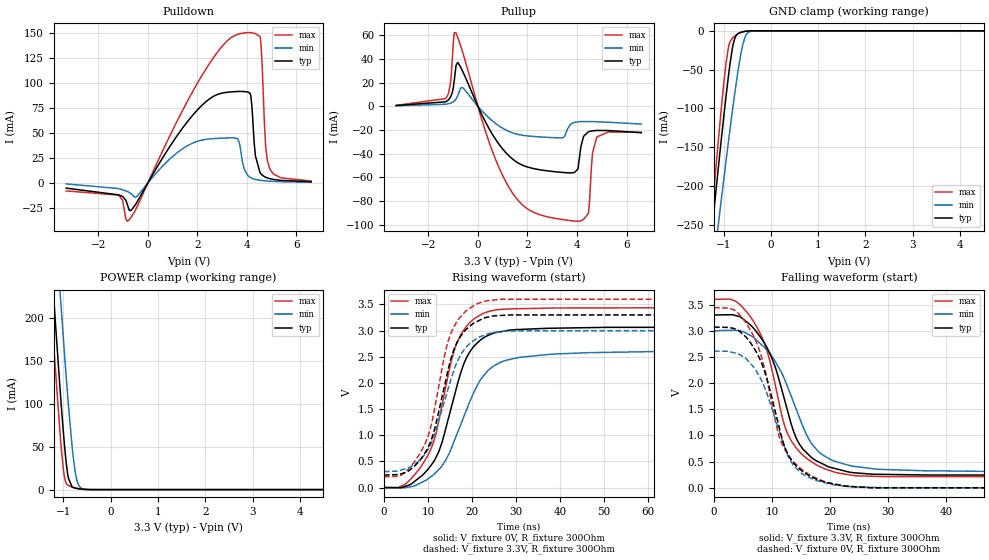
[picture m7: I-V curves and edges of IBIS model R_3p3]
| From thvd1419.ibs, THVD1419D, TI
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|   R_3p3 Model
[Model]   R_3p3
Model_type   3-state
Polarity   Non-Inverting
Vmeas = 1.65
Vref = 0
Cref = 2pF
Rref = 100000
|   typ   min   max
C_comp   4.717pF   4.609pF   4.761pF
| Where Nom  PVT is Nominal Process, 3.3V, 25C
|   Fast PVT is Strong Process,  3.6V, -40C
|   Slow PVT is Weak Process,   3.0V, 150C
[Voltage Range]   3.3   3   3.6
|Junction Temperature
[Temperature Range]   25   150   -40
[Pullup Reference]   3.3   3   3.6
[Pulldown Reference]   0   0   0
[Power Clamp Reference]   3.3   3   3.6
[GND Clamp Reference]   0   0   0
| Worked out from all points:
|   slope of the pulldown table from 0 to 0.495 V, typ, clamps not added: 23.7 ohm
|   slope of the pullup table from 0 to 0.495 V, typ, clamps not added: 24.1 ohm
|   GND clamp passes 1 mA (typ) near -0.58 V on its own axis
|   POWER clamp passes 1 mA (typ) near -0.67 V on its own axis
|   falling waveform, V_fixture 3.3V, R_fixture 300Ohm: 20-80 % time 5.55ns typ, 6.57ns min, 5.32ns max; typ from 3.3 V to 0.237 V
|   rising waveform, V_fixture 0V, R_fixture 300Ohm: 20-80 % time 6.58ns typ, 8.12ns min, 6.12ns max; typ from 0 V to 3.07 V
|   rising waveform, V_fixture 3.3V, R_fixture 300Ohm: 20-80 % time 5.67ns typ, 6.28ns min, 5.53ns max; typ from 0.237 V to 3.3 V
|   falling waveform, V_fixture 0V, R_fixture 300Ohm: 20-80 % time 4.96ns typ, 5.14ns min, 5.03ns max; typ from 3.07 V to 0 V
[Pulldown]
|   Voltage   I(typ)   I(min)   I(max)
-3.3V     -5.004mA   -808.9uA   -7.788mA
-1.191V   -11.72mA   -5.429mA   -11.96mA
-815.1mV  -22.29mA   -8.553mA   -38.1mA
2.373V    81.63mA    43.65mA    114.7mA
3.62V     91.29mA    44.25mA    148.2mA
4.046V    90.8mA     7.35mA     150mA
4.165V    85.92mA    5.258mA    149.9mA
4.343V    27.4mA     3.665mA    149mA
4.541V    10.13mA    2.745mA    145mA
4.759V    5.819mA    2.159mA    37.1mA
4.927V    4.383mA    1.859mA    14.12mA
6.6V      1.371mA    840.4uA    2.04mA
[GND Clamp]
|   Voltage   I(typ)   I(min)   I(max)
-3.3V     -1.553A    -1.424A    -1.755A
-1.379V   -339.1mA   -389.3mA   -331.1mA
-1.221V   -242.6mA   -306.6mA   -218.2mA
-1.112V   -177.7mA   -250.6mA   -143mA
-993.3mV  -109.4mA   -190.5mA   -66.79mA
-894.3mV  -57.17mA   -141.8mA   -20.64mA
-815.1mV  -23.4mA    -104.4mA   -9.506mA
-775.5mV  -12.37mA   -86.35mA   -7.293mA
-646.8mV  -2.133mA   -34.28mA   -2.532mA
-528mV    -536.9uA   -5.945mA   -571uA
-359.7mV  -25.12uA   -169.1uA   -14.99uA
6.6V      0A         0A         0A
[Pullup]
|   Voltage   I(typ)   I(min)   I(max)
-3.3V     632.8uA    409.7uA    833.3uA
-1.29V    4.001mA    1.824mA    6.974mA
-1.102V   7.96mA     2.751mA    20.36mA
-953.7mV  22.11mA    4.47mA     62.39mA
-884.4mV  34.56mA    6.104mA    62.1mA
-617.1mV  29.65mA    15.65mA    45.87mA
1.264V    -42.14mA   -21.34mA   -68.96mA
3.897V    -56.02mA   -13.6mA    -97.09mA
4.452V    -21.69mA   -12.87mA   -91.02mA
4.63V     -20.73mA   -12.96mA   -39.26mA
4.808V    -20.42mA   -13.08mA   -25.87mA
6.6V      -22.29mA   -15.03mA   -22.07mA
[POWER Clamp]
|   Voltage   I(typ)   I(min)   I(max)
-3.3V     2.079A     2.185A     2.031A
-1.449V   432.3mA    547.8mA    378.6mA
-1.251V   263.9mA    379.9mA    209.6mA
-1.221V   239.2mA    355.2mA    184.9mA
-1.191V   214.8mA    330.6mA    160.5mA
-1.063V   113mA      226.2mA    61.48mA
-983.4mV  57.32mA    164.8mA    17.27mA
-894.3mV  13.78mA    100.3mA    4.717mA
-805.2mV  2.832mA    45.77mA    2.884mA
-735.9mV  1.584mA    16.99mA    1.898mA
-567.6mV  338.7uA    707.7uA    328.3uA
6.6V      0A         0A         0A
[Ramp]
R_load = 300
|   typ   min   max
dV/dt_r   1.84126/6.54991e-09   1.56569/8.11927e-09   2.06375/6.11002e-09
dV/dt_f   1.83723/5.55202e-09   1.61722/6.53576e-09   2.0352/5.31971e-09
[Falling Waveform]
V_fixture = 3.3V
V_fixture_min = 3V
V_fixture_max = 3.6V
R_fixture = 300Ohm
C_fixture = 0F
|   Time   V(typ)   V(min)   V(max)
0s        3.3V       3V         3.599V
3.765ns   3.288V     3.008V     3.559V
7.362ns   2.97V      2.815V     3.072V
8.817ns   2.736V     2.665V     2.713V
10.41ns   2.346V     2.434V     2.029V
12.22ns   1.649V     2.051V     1.164V
14.01ns   987.4mV    1.54V      781.7mV
17.87ns   502.8mV    702.8mV    424.9mV
24.31ns   286.7mV    408.5mV    232mV
600ns     237.5mV    304.3mV    207.4mV
[Rising Waveform]
V_fixture = 0V
V_fixture_min = 0V
V_fixture_max = 0V
R_fixture = 300Ohm
C_fixture = 0F
|   Time   V(typ)   V(min)   V(max)
0s        474.2uV    405.4uV    533.1uV
7.695ns   166.8mV    60.46mV    318.5mV
10.56ns   410mV      200.2mV    714.8mV
12.5ns    697.2mV    346.4mV    1.289V
15.4ns    1.559V     767.2mV    2.447V
17.49ns   2.202V     1.212V     2.923V
22.13ns   2.831V     2.085V     3.308V
26.77ns   2.98V      2.402V     3.405V
66.42ns   3.06V      2.602V     3.434V
600ns     3.069V     2.61V      3.44V
[Rising Waveform]
V_fixture = 3.3V
V_fixture_min = 3V
V_fixture_max = 3.6V
R_fixture = 300Ohm
C_fixture = 0F
|   Time   V(typ)   V(min)   V(max)
0s        237.5mV    304.3mV    207.4mV
4.66ns    282.9mV    352.8mV    281.9mV
9.212ns   646.8mV    628.6mV    814.9mV
10.39ns   830.8mV    785.9mV    1.078V
11.47ns   1.103V     1.011V     1.486V
14.25ns   2.126V     1.792V     2.694V
16.59ns   2.768V     2.391V     3.171V
19.94ns   3.112V     2.783V     3.448V
26.77ns   3.288V     2.983V     3.597V
600ns     3.3V       3V         3.599V
[Falling Waveform]
|Gnd
V_fixture = 0V
V_fixture_min = 0V
V_fixture_max = 0V
R_fixture = 300Ohm
C_fixture = 0F
|   Time   V(typ)   V(min)   V(max)
0s        3.069V     2.61V      3.44V
3.462ns   3.041V     2.577V     3.397V
6.557ns   2.722V     2.339V     2.953V
8.624ns   2.248V     1.938V     2.314V
11.2ns    1.16V      1.091V     988.2mV
12.31ns   738.2mV    731.4mV    706.9mV
13.61ns   488mV      439.3mV    508.9mV
18.96ns   115.5mV    102.6mV    122.2mV
26.77ns   6.16mV     10.21mV    1.985mV
600ns     474.2uV    405.4uV    533.1uV
